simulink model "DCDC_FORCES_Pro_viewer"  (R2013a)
settings: Solver=ode45  StartTime=0.0  StopTime=8e-3  RelTol=1e-3
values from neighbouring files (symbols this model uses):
  Ad = Pd.a    [DCDCConverter.m]
  Bd1 = Bd(:,1)    [DCDCConverter.m]
  Bd2 = Bd(:,2:3)    [DCDCConverter.m]
  Cd2 = Cd(3,:)    [DCDCConverter.m]
  Dd3 = Dd(3,1)    [DCDCConverter.m]
  Dd4 = Dd(3,2:3)    [DCDCConverter.m]
  Q = [.01, 0; 0, 10]    [DCDCConverter.m]
  R = 1    [DCDCConverter.m]
undefined symbols (not defined in the file or in its folder): plecs

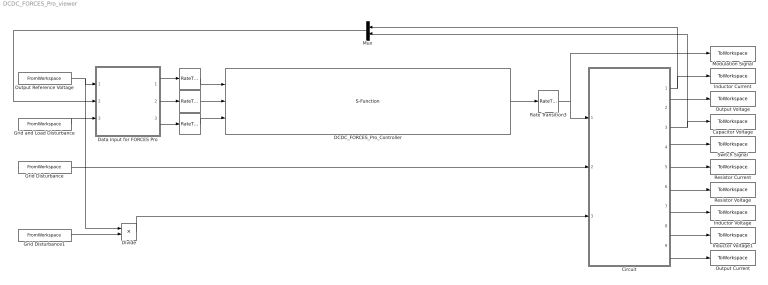
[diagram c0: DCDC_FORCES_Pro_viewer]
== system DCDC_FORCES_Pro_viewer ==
  " " : RateTransition  OutPortSampleTime=T_control
  "  " : RateTransition  OutPortSampleTime=T_control
  "   " : RateTransition  OutPortSampleTime=T_control
  Capacitor Voltage : ToWorkspace  VariableName=u_C_MPCPlecs  SampleTime=-1  SaveFormat=Timeseries
  Circuit : Subsystem  LoadFcn=plecs('sl', 200);  InitFcn=plecs('sl', 214);  StartFcn=plecs('sl', 208);  StopFcn=plecs('sl', 209);
  DCDC_FORCES_Pro_Controller : S-Function  FunctionName=DCDC_FORCES_Pro_Controller_simulinkBlock  EnableBusSupport=off
  Data Input for FORCES Pro : Subsystem
  Divide : Product  Inputs=*/
  Grid Disturbance : FromWorkspace  VariableName=[t, Grid_Dist_PL]  SampleTime=0
  Grid Disturbance1 : FromWorkspace  VariableName=[t, Load_Dist_PL]  SampleTime=0
  Grid and Load Disturbance : FromWorkspace  VariableName=[t, w']  SampleTime=0
  Inductor Current : ToWorkspace  VariableName=i_L_MPCPlecs  SampleTime=-1  SaveFormat=Timeseries
  Inductor Voltage : ToWorkspace  VariableName=u_L_MPCPlecs  SampleTime=-1  SaveFormat=Timeseries
  Inductor Voltage1 : ToWorkspace  VariableName=i_IN_MPCPlecs  SampleTime=-1  SaveFormat=Timeseries
  Modulation Signal : ToWorkspace  VariableName=m_MPCPlecs  SampleTime=-1  SaveFormat=Timeseries
  Mux : Mux  Inputs=2
  Output Current : ToWorkspace  VariableName=i_OUT_MPCPlecs  SampleTime=-1  SaveFormat=Timeseries
  Output Reference Voltage : FromWorkspace  VariableName=[t, U_out_ref]  SampleTime=0
  Output Voltage : ToWorkspace  VariableName=U_out_MPCPlecs  SampleTime=-1  SaveFormat=Timeseries
  Rate Transition3 : RateTransition  OutPortSampleTime=T_control
  Resistor Current : ToWorkspace  VariableName=i_R_MPCPlecs  SampleTime=-1  SaveFormat=Timeseries
  Resistor Voltage : ToWorkspace  VariableName=u_R_MPCPlecs  SampleTime=-1  SaveFormat=Timeseries
  Switch Signal : ToWorkspace  VariableName=d_MPCPlecs  SampleTime=-1  SaveFormat=Timeseries
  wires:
  Circuit/2(U out) -> Output Voltage/1
  Circuit/3(u C) -> Capacitor Voltage/1, Mux/2
  Circuit/1(i L) -> Inductor Current/1, Mux/1
  DCDC_FORCES_Pro_Controller/1 -> Rate Transition3/1
  Circuit/4(d) -> Switch Signal/1
  Grid and Load Disturbance/1 -> Data Input for FORCES Pro/3(Disturbance)
  Output Reference Voltage/1 -> Divide/1, Data Input for FORCES Pro/1(U_out_ref)
  Mux/1 -> Data Input for FORCES Pro/2(states)
  Data Input for FORCES Pro/1(mAmB) -> "  "/1
  Data Input for FORCES Pro/2(LT) -> " "/1
  Data Input for FORCES Pro/3(B2w) -> "   "/1
  "  "/1 -> DCDC_FORCES_Pro_Controller/1
  " "/1 -> DCDC_FORCES_Pro_Controller/2
  "   "/1 -> DCDC_FORCES_Pro_Controller/3
  Rate Transition3/1 -> Modulation Signal/1, Circuit/1(Mod Signal)
  Circuit/5(i R) -> Resistor Current/1
  Circuit/6(u R) -> Resistor Voltage/1
  Circuit/7(u L) -> Inductor Voltage/1
  Circuit/8(i IN) -> Inductor Voltage1/1
  Circuit/9(i OUT) -> Output Current/1
  Grid Disturbance/1 -> Circuit/2(Grid Voltage)
  Divide/1 -> Circuit/3(Load Resistance)
  Grid Disturbance1/1 -> Divide/2

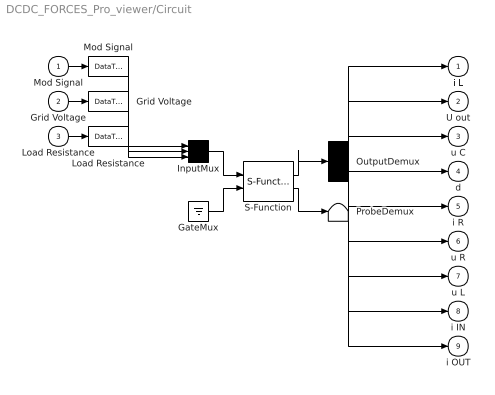
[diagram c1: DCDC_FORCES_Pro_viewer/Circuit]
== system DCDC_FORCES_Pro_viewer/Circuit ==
  Mod Signal : Inport  PortDimensions=1
  Grid Voltage : Inport  Port=2  PortDimensions=1
  Load Resistance : Inport  Port=3  PortDimensions=1
  " GateMux " : Ground
  " Grid Voltage " : DataTypeConversion
  " InputMux " : Mux  Inputs=[ 1 1 1 ]
  " Load Resistance " : DataTypeConversion
  " Mod Signal " : DataTypeConversion
  " OutputDemux " : Demux  Outputs=[ 1 1 1 1 1 1 1 1 1 ]
  " ProbeDemux " : Terminator
  " S-Function " : S-Function  FunctionName=plecs  EnableBusSupport=off
  i L : Outport  PortDimensions=1
  U out : Outport  Port=2  PortDimensions=1
  u C : Outport  Port=3  PortDimensions=1
  d : Outport  Port=4  PortDimensions=1
  i R : Outport  Port=5  PortDimensions=1
  u R : Outport  Port=6  PortDimensions=1
  u L : Outport  Port=7  PortDimensions=1
  i IN : Outport  Port=8  PortDimensions=1
  i OUT : Outport  Port=9  PortDimensions=1
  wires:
  " S-Function "/1 -> " OutputDemux "/1
  " InputMux "/1 -> " S-Function "/1
  " GateMux "/1 -> " S-Function "/2
  " S-Function "/2 -> " ProbeDemux "/1
  Mod Signal/1 -> " Mod Signal "/1
  " Mod Signal "/1 -> " InputMux "/1
  Grid Voltage/1 -> " Grid Voltage "/1
  " Grid Voltage "/1 -> " InputMux "/2
  Load Resistance/1 -> " Load Resistance "/1
  " Load Resistance "/1 -> " InputMux "/3
  " OutputDemux "/1 -> i L/1
  " OutputDemux "/2 -> U out/1
  " OutputDemux "/3 -> u C/1
  " OutputDemux "/4 -> d/1
  " OutputDemux "/5 -> i R/1
  " OutputDemux "/6 -> u R/1
  " OutputDemux "/7 -> u L/1
  " OutputDemux "/8 -> i IN/1
  " OutputDemux "/9 -> i OUT/1

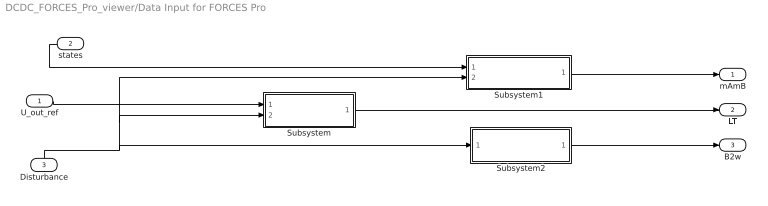
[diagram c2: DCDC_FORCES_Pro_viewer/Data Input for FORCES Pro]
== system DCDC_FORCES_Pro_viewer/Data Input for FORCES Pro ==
  U_out_ref : Inport
  states : Inport  Port=2
  Disturbance : Inport  Port=3
  Subsystem : Subsystem
  Subsystem1 : Subsystem
  Subsystem2 : Subsystem
  mAmB : Outport
  LT : Outport  Port=2
  B2w : Outport  Port=3
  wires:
  U_out_ref/1 -> Subsystem/1(U_out_ref)
  Subsystem/1(Linear Term) -> LT/1
  states/1 -> Subsystem1/1(states)
  Subsystem2/1(B2w) -> B2w/1
  Subsystem1/1(mAmB) -> mAmB/1
  Disturbance/1 -> Subsystem2/1(Distrubances), Subsystem/2(Disturbances), Subsystem1/2(Disturbance)

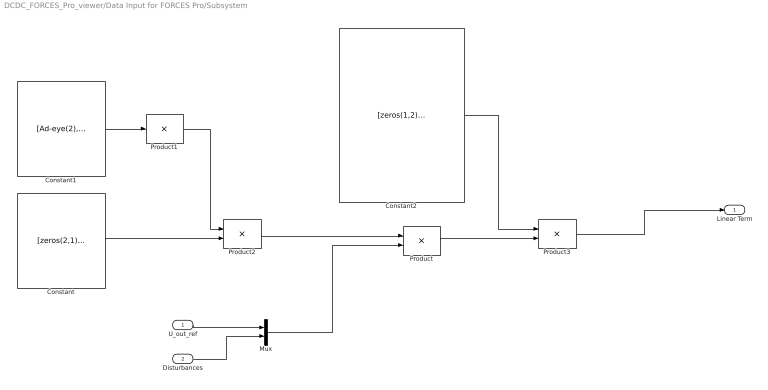
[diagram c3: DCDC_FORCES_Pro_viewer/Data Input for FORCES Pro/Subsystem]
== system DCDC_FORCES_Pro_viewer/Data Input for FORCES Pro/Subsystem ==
  U_out_ref : Inport
  Disturbances : Inport  Port=2
  Constant : Constant  Value=[zeros(2,1), -Bd2; 1, -Dd4]
  Constant1 : Constant  Value=[Ad-eye(2), Bd1; Cd2, Dd3]
  Constant2 : Constant  Value=[zeros(1,2), -R; -Q,zeros(2,1)]
  Mux : Mux  Inputs=2
  Product : Product  Inputs=**  Multiplication=Matrix(*)  SampleTime=1e-7
  Product1 : Product  Inputs=/  Multiplication=Matrix(*)  SampleTime=1e-7
  Product2 : Product  Inputs=**  Multiplication=Matrix(*)  SampleTime=1e-7
  Product3 : Product  Inputs=**  Multiplication=Matrix(*)  SampleTime=1e-7
  Linear Term : Outport
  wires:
  Disturbances/1 -> Mux/2
  U_out_ref/1 -> Mux/1
  Product1/1 -> Product2/1
  Constant1/1 -> Product1/1
  Constant/1 -> Product2/2
  Product2/1 -> Product/1
  Product3/1 -> Linear Term/1
  Constant2/1 -> Product3/1
  Product/1 -> Product3/2
  Mux/1 -> Product/2

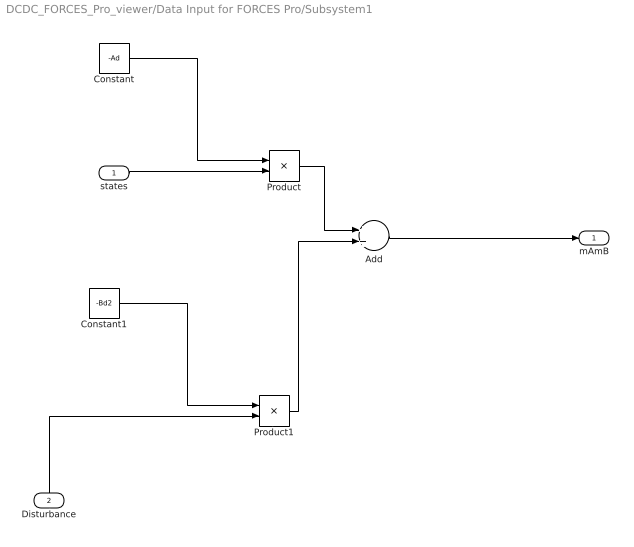
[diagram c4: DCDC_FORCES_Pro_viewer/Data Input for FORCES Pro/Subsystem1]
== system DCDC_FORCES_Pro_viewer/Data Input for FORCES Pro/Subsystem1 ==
  states : Inport
  Disturbance : Inport  Port=2
  Add : Sum  SampleTime=1e-7
  Constant : Constant  Value=-Ad
  Constant1 : Constant  Value=-Bd2
  Product : Product  Inputs=**  Multiplication=Matrix(*)  SampleTime=1e-7
  Product1 : Product  Inputs=**  Multiplication=Matrix(*)  SampleTime=1e-7
  mAmB : Outport
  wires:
  states/1 -> Product/2
  Add/1 -> mAmB/1
  Constant/1 -> Product/1
  Product/1 -> Add/1
  Constant1/1 -> Product1/1
  Disturbance/1 -> Product1/2
  Product1/1 -> Add/2

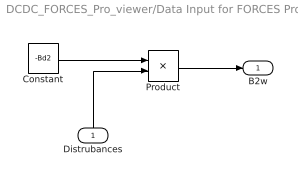
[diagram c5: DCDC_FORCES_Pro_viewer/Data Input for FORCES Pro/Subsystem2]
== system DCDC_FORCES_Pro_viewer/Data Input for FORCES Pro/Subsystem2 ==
  Distrubances : Inport
  Constant : Constant  Value=-Bd2
  Product : Product  Inputs=**  Multiplication=Matrix(*)  SampleTime=1e-7
  B2w : Outport
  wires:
  Product/1 -> B2w/1
  Distrubances/1 -> Product/2
  Constant/1 -> Product/1
